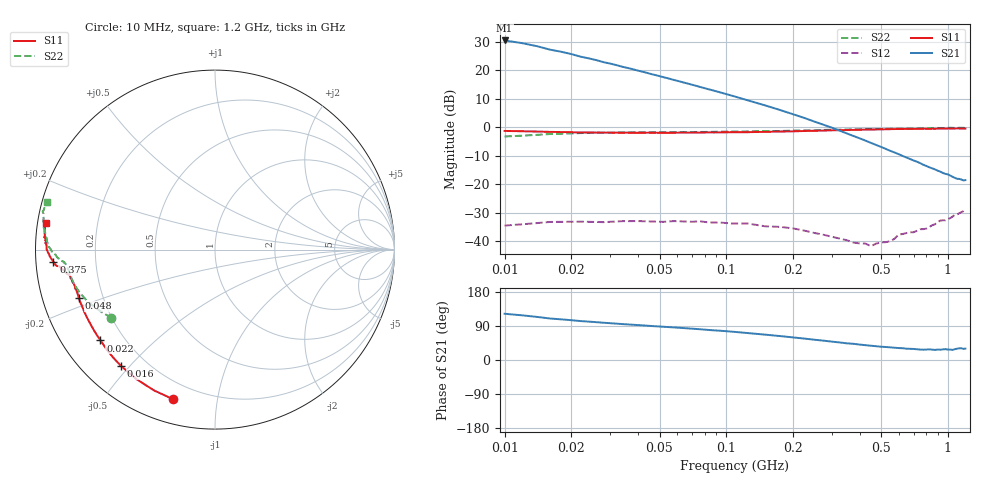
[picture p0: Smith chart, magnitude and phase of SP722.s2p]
!  POLYFET RF DEVICES
!  S PARAMETERS FOR
!  SP722
!  VDS=12.5, IDQ=400MA
# MHZ  S  MA  R  50.0000
! SCATTERING PARAMETERS :
! Freq=MHz Mag[s11] Ang[s11] Mag[s21] Ang[s21] Mag[s12] Ang[s12] Mag[s22] Ang[s22]
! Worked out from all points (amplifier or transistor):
!   95 points, 10 MHz to 1.2 GHz, reference 50 ohm
!   highest |S21| = 30.5 dB at 10 MHz (marker M1)
!   |S21| within 3 dB of that: start of sweep to 15.64 MHz
!   unconditionally stable (mu >= 1): 308.6 MHz to end of sweep
!   at 40 MHz: K = 0.11, MSG = 26.4 dB, |S12| = -32.9 dB
!   at 104 MHz: K = 0.26, MSG = 22.5 dB, |S12| = -33.7 dB
!   at 1.2 GHz: K = 1.24, MAG = 2.3 dB, |S12| = -29.0 dB
!   S11 on the Smith chart (normalised r, x): 10 MHz: 0.11, -0.75; 16 MHz: 0.11, -0.47; 22 MHz: 0.11, -0.34; 48 MHz: 0.11, -0.17; 375 MHz: 0.05, -0.04; 1.2 GHz: 0.02, +0.08
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10  0.8657 -105.7  33.67 122.0  0.0188 32.2  0.6907 -146.6
12  0.8549 -113.5  30.19 117.9  0.01979 28.5  0.7148 -150.2
14  0.8441 -121.2  26.72 113.7  0.02079 24.8  0.7389 -153.8
16  0.8333 -129.0  23.24 109.6  0.02178 21.1  0.7631 -157.3
18  0.827 -133.2  21.32 107.3  0.02186 18.7  0.7732 -159.2
20  0.8207 -137.4  19.4 105.0  0.02194 16.2  0.7833 -161.1
22  0.8144 -141.6  17.48 102.8  0.02202 13.8  0.7934 -162.9
24  0.8124 -144.0  16.31 101.3  0.02188 12.9  0.7982 -164.0
28  0.8085 -148.9  13.97 98.3  0.0216 11.0  0.8077 -166.1
34  0.8066 -154.2  11.61 94.7  0.02249 8.8  0.8149 -168.4
40  0.8047 -157.3  9.922 92.1  0.02254 6.5  0.8185 -170.3
48  0.8053 -160.6  8.284 89.0  0.02208 2.5  0.8224 -171.3
50  0.8046 -161.2  7.956 88.4  0.02198 2.3  0.8228 -171.6
58  0.8043 -163.5  6.813 86.0  0.02253 0.2  0.8265 -172.6
76  0.8101 -166.4  5.145 81.2  0.02236 -3.1  0.831 -173.8
110  0.8202 -169.4  3.459 74.0  0.02042 -5.8  0.8447 -175.1
125  0.8229 -170.0  2.987 71.1  0.02044 -8.0  0.8488 -175.6
175  0.8443 -171.6  2.018 63.1  0.01784 -11.8  0.8646 -176.5
250  0.871 -173.8  1.264 53.5  0.01393 -9.3  0.8882 -178.2
375  0.9029 -175.7  0.705 42.7  0.00945 4.7  0.9245 179.1
550  0.9297 -178.8  0.3863 33.4  0.01001 54.3  0.9462 175.5
1200  0.9551 171.1  0.1181 30.2  0.03559 83.7  0.9738 164.3
